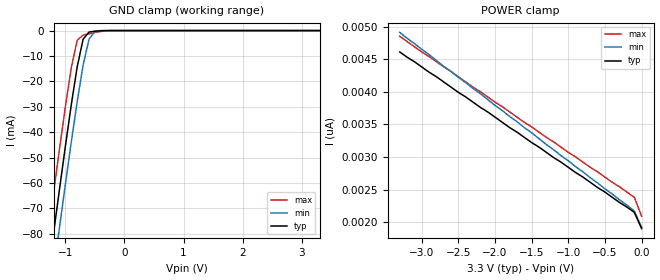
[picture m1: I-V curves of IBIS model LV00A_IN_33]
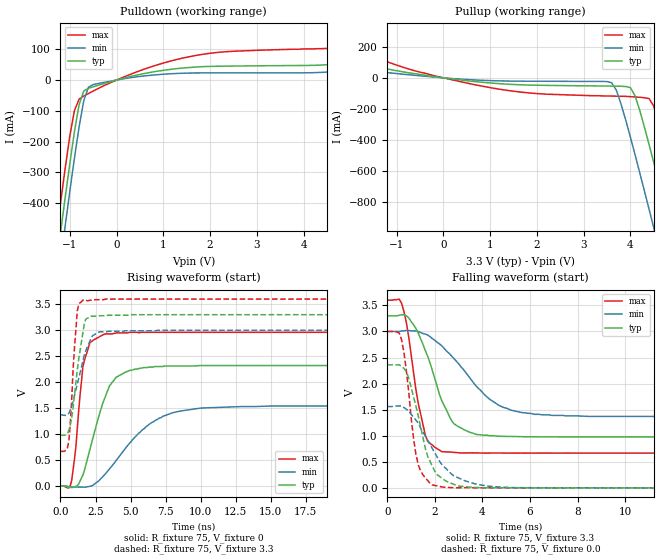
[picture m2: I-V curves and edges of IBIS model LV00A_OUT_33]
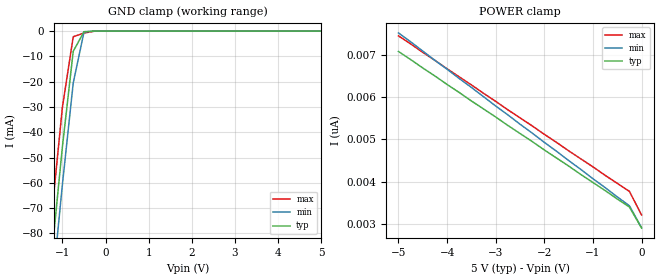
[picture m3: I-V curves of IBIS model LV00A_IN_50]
| TEXAS INSTRUMENTS INCORPORATED
| Standard Linear and Logic Group
| IBIS Model of SN74LV00A
| QUADRUPLE 2-INPUT POSITIVE-NAND GATE
| SOIC 14-pin (D), SOP 14-pin (NS), SSOP 14-pin (DB), TSSOP 14-pin (PW)
| and TVSOP 14-pin (DGV) Package
[IBIS Ver]   3.2
[Comment Char]  |_char
[File Name]   lv00a.ibs
[File Rev]   2.0 I_die
[Date]   May 26, 2000
[Source]   Data created from HSPICE simulations at TI-SLL.
[Notes]   The following is an IBIS list for the LV00A.
|   Please contact sllibis@ti.com with questions and
|   comments concerning SLL IBIS models.
[Disclaimer] Property of Texas Instruments Incorporated.  Unauthorized
   reproduction and/or distribution is strictly prohibited.
   This product is protected under copyright law.
   Created 2000, (C) Copyright 2000, Texas Instruments Inc.,
   All Rights Reserved.
   UNLESS THERE IS A SIGNED, WRITTEN AGREEMENT TO THE
   CONTRARY, TEXAS INSTRUMENTS () IS PROVIDING THE IBIS
   MODELS  AND WITHOUT ANY WARRANTY, EXPRESSED OR
   IMPLIED.  TI assumes no liability for:
   1) the accuracy of the IBIS models provided to your
   company;
   2) the proper functioning of these IBIS Models in your
   design or for any resulting applications; or
   3) infringement of patents, copyrights or intellectual
   property rights resulting from your use of these IBIS
   models.
   TI provides IBIS Models as a service to our customers.
   You and your company shall not distribute, sell or give
   these models to anyone else without prior written
   permission from TI.
   TI reserves the right to make changes to our products or
   to discontinue any semiconductor product or service
   without notice, and advises our customers to obtain the
   latest version of relevant information to verify, before
   placing orders, that the information being relied on is
   current.
   Please be aware that your receipt and use of the IBIS
   information provided shall serve as acceptance of these
   terms and conditions.  If you do not accept these terms,
   you should return or destroy the IBIS models and any
   other accompanying information immediately.
|   Component LV00A_D
[Component]   LV00A_D
[Manufacturer]  Texas Instruments, Inc.
[Package]
|   typ   min   max
R_pkg   0.031   0.028   0.034
L_pkg   3.109nH   2.462nH   3.889nH
C_pkg   0.473pF   0.363pF   0.628pF
[Pin]   signal_name   model_name   R_pin   L_pin   C_pin
1   1A   LV00A_IN   0.033   3.854nH   0.622pF
2   1B   LV00A_IN   0.032   3.188nH   0.473pF
3   1Y   LV00A_OUT   0.028   2.462nH   0.377pF
4   2A   LV00A_IN   0.031   2.596nH   0.363pF
5   2B   LV00A_IN   0.028   2.521nH   0.372pF
6   2Y   LV00A_OUT   0.034   3.250nH   0.476pF
7   GND   GND   0.034   3.889nH   0.628pF
8   3Y   LV00A_OUT   0.034   3.889nH   0.628pF
9   3A   LV00A_IN   0.034   3.250nH   0.476pF
10   3B   LV00A_IN   0.028   2.521nH   0.372pF
11   4Y   LV00A_OUT   0.031   2.596nH   0.364pF
12   4A   LV00A_IN   0.028   2.462nH   0.377pF
13   4B   LV00A_IN   0.032   3.188nH   0.473pF
14   VCC   POWER   0.033   3.854nH   0.622pF
|   Component LV00A_NS
[Component]   LV00A_NS
[Manufacturer]  Texas Instruments, Inc.
[Package]
|   typ   min   max
R_pkg   0.045   0.039   0.054
L_pkg   3.796nH   2.561nH   4.952nH
C_pkg   0.528pF   0.288pF   0.710pF
[Pin]   signal_name   model_name   R_pin   L_pin   C_pin
1   1A   LV00A_IN   0.047   4.867nH   0.706pF
2   1B   LV00A_IN   0.051   4.083nH   0.592pF
3   1Y   LV00A_OUT   0.041   2.915nH   0.376pF
4   2A   LV00A_IN   0.039   2.561nH   0.288pF
5   2B   LV00A_IN   0.041   3.101nH   0.430pF
6   2Y   LV00A_OUT   0.047   4.047nH   0.589pF
7   GND   GND   0.051   4.909nH   0.700pF
8   3Y   LV00A_OUT   0.045   4.784nH   0.694pF
9   3A   LV00A_IN   0.054   4.176nH   0.597pF
10   3B   LV00A_IN   0.039   3.287nH   0.449pF
11   4Y   LV00A_OUT   0.039   2.586nH   0.294pF
12   4A   LV00A_IN   0.040   2.802nH   0.371pF
13   4B   LV00A_IN   0.049   4.080nH   0.593pF
14   VCC   POWER   0.052   4.952nH   0.710pF
|   Component LV00A_DB
[Component]   LV00A_DB
[Manufacturer]  Texas Instruments, Inc.
[Package]
|   typ   min   max
R_pkg   0.044   0.041   0.046
L_pkg   3.551nH   3.258nH   3.927nH
C_pkg   0.402pF   0.360pF   0.421pF
[Pin]   signal_name   model_name   R_pin   L_pin   C_pin
1   1A   LV00A_IN   0.046   3.927nH   0.408pF
2   1B   LV00A_IN   0.044   3.587nH   0.421pF
3   1Y   LV00A_OUT   0.041   3.289nH   0.398pF
4   2A   LV00A_IN   0.042   3.258nH   0.360pF
5   2B   LV00A_IN   0.041   3.286nH   0.403pF
6   2Y   LV00A_OUT   0.044   3.586nH   0.421pF
7   GND   GND   0.046   3.927nH   0.408pF
8   3Y   LV00A_OUT   0.046   3.927nH   0.408pF
9   3A   LV00A_IN   0.044   3.586nH   0.421pF
10   3B   LV00A_IN   0.041   3.286nH   0.403pF
11   4Y   LV00A_OUT   0.043   3.258nH   0.360pF
12   4A   LV00A_IN   0.041   3.289nH   0.398pF
13   4B   LV00A_IN   0.044   3.587nH   0.421pF
14   VCC   POWER   0.046   3.927nH   0.408pF
|   Component LV00A_PW
[Component]   LV00A_PW
[Manufacturer]  Texas Instruments, Inc.
[Package]
|   typ   min   max
R_pkg   0.032   0.029   0.035
L_pkg   2.378nH   2.170nH   2.680nH
C_pkg   0.314pF   0.270pF   0.335pF
[Pin]   signal_name   model_name   R_pin   L_pin   C_pin
1   1A   LV00A_IN   0.033   2.618nH   0.330pF
2   1B   LV00A_IN   0.031   2.313nH   0.317pF
3   1Y   LV00A_OUT   0.030   2.310nH   0.314pF
4   2A   LV00A_IN   0.031   2.173nH   0.272pF
5   2B   LV00A_IN   0.030   2.204nH   0.309pF
6   2Y   LV00A_OUT   0.032   2.315nH   0.317pF
7   GND   GND   0.035   2.680nH   0.335pF
8   3Y   LV00A_OUT   0.033   2.640nH   0.333pF
9   3A   LV00A_IN   0.034   2.347nH   0.319pF
10   3B   LV00A_IN   0.029   2.277nH   0.313pF
11   4Y   LV00A_OUT   0.031   2.170nH   0.270pF
12   4A   LV00A_IN   0.031   2.244nH   0.311pF
13   4B   LV00A_IN   0.033   2.343nH   0.321pF
14   VCC   POWER   0.035   2.657nH   0.332pF
|   Component LV00A_DGV
[Component]   LV00A_DGV
[Manufacturer]  Texas Instruments, Inc.
[Package]
|   typ   min   max
R_pkg   0.035   0.020   0.045
L_pkg   2.499nH   2.077nH   2.966nH
C_pkg   0.361pF   0.305pF   0.416pF
[Pin]   signal_name   model_name   R_pin   L_pin   C_pin
1   1A   LV00A_IN   0.027   2.717nH   0.373pF
2   1B   LV00A_IN   0.037   2.434nH   0.398pF
3   1Y   LV00A_OUT   0.034   2.200nH   0.316pF
4   2A   LV00A_IN   0.020   2.077nH   0.309pF
5   2B   LV00A_IN   0.030   2.147nH   0.305pF
6   2Y   LV00A_OUT   0.042   2.580nH   0.408pF
7   GND   GND   0.039   2.921nH   0.385pF
8   3Y   LV00A_OUT   0.033   2.841nH   0.380pF
9   3A   LV00A_IN   0.042   2.611nH   0.410pF
10   3B   LV00A_IN   0.038   2.331nH   0.329pF
11   4Y   LV00A_OUT   0.026   2.223nH   0.319pF
12   4A   LV00A_IN   0.034   2.259nH   0.313pF
13   4B   LV00A_IN   0.045   2.681nH   0.416pF
14   VCC   POWER   0.042   2.966nH   0.386pF
[Model Selector]   LV00A_IN
LV00A_IN_33   3.3-V Vcc Input Model
LV00A_IN_50   5.0-V Vcc Input Model
[Model Selector]   LV00A_OUT
LV00A_OUT_33   3.3-V Vcc Output Model
LV00A_OUT_50   5.0-V Vcc Output Model
| Models and submodels in the file (4): LV00A_IN_33 (Input), LV00A_OUT_33 (Output), LV00A_IN_50 (Input), LV00A_OUT_50 (Output)
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|   Model LV00A_IN_33
[Model]   LV00A_IN_33
Model_type  Input
Polarity   Inverting
Vinl = 0.99
Vinh = 2.31
| variable   typ   min   max
C_comp   1.24pf   0.94pf   1.54pf
[Temperature Range]   25   85   -40
[Voltage Range]   3.3   3.0   3.6
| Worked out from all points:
|   GND clamp passes 1 mA (typ) near -0.61 V on its own axis
[GND Clamp]
|   Voltage   I(typ)   I(min)   I(max)
-3.3V     -460mA     -475mA     -445mA
-1.3V     -97.5mA    -113mA     -81.5mA
-1.2V     -79.9mA    -95mA      -63.9mA
-1.1V     -62.6mA    -77.6mA    -46.7mA
-1V       -45.6mA    -60.5mA    -30mA
-900mV    -29.2mA    -43.9mA    -14.6mA
-800mV    -14.3mA    -28mA      -3.81mA
-700mV    -3.42mA    -13.6mA    -1.78mA
-600mV    -581uA     -3.4mA     -1.25mA
-500mV    -233uA     -353uA     -759uA
-400mV    -58.1uA    -21.9uA    -324uA
3.3V      1.9nA      2.34nA     1.69nA
[POWER Clamp]
|   Voltage   I(typ)   I(min)   I(max)
-3.3V     4.61nA     4.91nA     4.85nA
-3V       4.38nA     4.65nA     4.61nA
-100mV    2.15nA     2.17nA     2.38nA
0V        1.9nA      1.92nA     2.09nA
|   Model LV00A_OUT_33
[Model]   LV00A_OUT_33
Model_type  Output
Polarity   Non-Inverting
Vmeas = 1.65v
Cref = 15pf
| variable   typ   min   max
C_comp   4.62pf   3.47pf   5.77pf
[Temperature Range]   25   85   -40
[Voltage Range]   3.3   3.0   3.6
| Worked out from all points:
|   slope of the pulldown table from 0 to 0.495 V, typ, clamps not added: 27.3 ohm
|   slope of the pullup table from 0 to 0.495 V, typ, clamps not added: 27.2 ohm
|   rising waveform, R_fixture 75, V_fixture 0: 20-80 % time 1.52ns typ, 3.17ns min, 629ps max; typ from 0 V to 2.32 V
|   falling waveform, R_fixture 75, V_fixture 3.3: 20-80 % time 1.12ns typ, 1.92ns min, 624ps max; typ from 3.3 V to 0.976 V
|   rising waveform, R_fixture 75, V_fixture 3.3: 20-80 % time 664ps typ, 943ps min, 389ps max; typ from 0.976 V to 3.3 V
|   falling waveform, R_fixture 75, V_fixture 0.0: 20-80 % time 811ps typ, 1.31ns min, 468ps max; typ from 2.36 V to 0 V
[Pulldown]
|   Voltage   I(typ)   I(min)   I(max)
-3.3V     -3.04A     -3.13A     -2.95A
-1.3V     -615mA     -707mA     -518mA
-1.2V     -498mA     -591mA     -401mA
-1.1V     -383mA     -475mA     -288mA
-900mV    -167mA     -253mA     -98.6mA
-800mV    -79.1mA    -151mA     -61.7mA
-700mV    -35.5mA    -66.4mA    -51.9mA
-600mV    -26.8mA    -23.2mA    -43.9mA
-500mV    -22mA      -14.7mA    -35.8mA
1.6V      41.2mA     22.8mA     77.1mA
4.7V      52.1mA     27.5mA     106mA
6.6V      86.8mA     47.3mA     166mA
[Pullup]
|   Voltage   I(typ)   I(min)   I(max)
-3.3V     168mA      92.9mA     314mA
600mV     -21.6mA    -12.3mA    -39.7mA
3.6V      -52.9mA    -31.5mA    -117mA
3.8V      -54.2mA    -168mA     -119mA
4V        -62.6mA    -381mA     -121mA
4.1V      -115mA     -494mA     -123mA
4.4V      -429mA     -845mA     -133mA
4.5V      -544mA     -964mA     -182mA
4.8V      -899mA     -1.32A     -505mA
4.9V      -1.02A     -1.44A     -622mA
5.2V      -1.38A     -1.81A     -981mA
6.6V      -3.09A     -3.52A     -2.69A
[Ramp]
| variable   typ   min   max
dV/dt_r   1.39E+00/1.49E-09   9.32E-01/3.20E-09   1.78E+00/6.41E-10
dV/dt_f   1.41E+00/1.08E-09   9.91E-01/1.94E-09   1.77E+00/6.09E-10
R_load = 75
[Rising Waveform]
R_fixture = 75
V_fixture = 0
|   Time   V(typ)   V(min)   V(max)
0s        0V         0V         0V
800ps     -32.3mV    -18.1mV    101mV
1.6ns     209mV      -24.4mV    2.3V
1.7ns     290mV      -25.1mV    2.41V
2.1ns     701mV      -8.51mV    2.76V
3ns       1.58V      173mV      2.91V
3.5ns     1.93V      328mV      2.93V
4.6ns     2.19V      711mV      2.95V
8ns       2.31V      1.41V      2.96V
25ns      2.32V      1.54V      2.96V
[Falling Waveform]
R_fixture = 75
V_fixture = 3.3
V_fixture_min = 3.0
V_fixture_max = 3.6
|   Time   V(typ)   V(min)   V(max)
0s        3.3V       3V         3.6V
600ps     3.32V      3.01V      3.54V
1.1ns     3.13V      3.01V      2.22V
1.6ns     2.63V      2.95V      1.01V
2.3ns     1.66V      2.72V      693mV
2.8ns     1.23V      2.48V      681mV
3.5ns     1.06V      2.09V      672mV
4.7ns     991mV      1.58V      668mV
6.2ns     980mV      1.41V      666mV
25ns      976mV      1.37V      666mV
[Rising Waveform]
R_fixture = 75
V_fixture = 3.3
V_fixture_min = 3.0
V_fixture_max = 3.6
|   Time   V(typ)   V(min)   V(max)
0s        976mV      1.37V      666mV
600ps     1.07V      1.4V       864mV
800ps     1.31V      1.53V      1.64V
900ps     1.5V       1.62V      2.24V
1.2ns     2.23V      1.96V      3.37V
1.6ns     2.95V      2.41V      3.58V
1.8ns     3.21V      2.6V       3.58V
2.3ns     3.27V      2.9V       3.59V
2.8ns     3.28V      2.97V      3.59V
25ns      3.3V       3V         3.6V
[Falling Waveform]
R_fixture = 75
V_fixture = 0.0
|   Time   V(typ)   V(min)   V(max)
0s        2.36V      1.56V      3V
500ps     2.36V      1.57V      2.97V
600ps     2.33V      1.57V      2.84V
800ps     2.23V      1.51V      2.25V
1.2ns     1.57V      1.3V       650mV
1.6ns     752mV      992mV      193mV
1.9ns     410mV      748mV      55.3mV
2.8ns     66.6mV     231mV      2.1mV
4.7ns     2.69mV     16.1mV     545uV
25ns      9.56uV     0V         13.6uV
|   Model LV00A_IN_50
[Model]   LV00A_IN_50
Model_type  Input
Polarity   Inverting
Vinl = 1.5
Vinh = 3.5
| variable   typ   min   max
C_comp   1.24pf   0.94pf   1.54pf
[Temperature Range]   25   85   -40
[Voltage Range]   5.0   4.5   5.5
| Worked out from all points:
|   GND clamp passes 1 mA (typ) near -0.52 V on its own axis
[GND Clamp]
|   Voltage   I(typ)   I(min)   I(max)
-5V       -773mA     -786mA     -758mA
-1.5V     -133mA     -148mA     -117mA
-1.25V    -88.7mA    -104mA     -72.7mA
-1V       -45.6mA    -60.5mA    -30mA
-750mV    -7.99mA    -20.5mA    -2.23mA
-500mV    -233uA     -353uA     -759uA
-250mV    -2.63nA    -182nA     -26.9uA
5V        2.9nA      3.64nA     2.54nA
[POWER Clamp]
|   Voltage   I(typ)   I(min)   I(max)
-5V       7.08nA     7.52nA     7.45nA
-1.5V     4.37nA     4.5nA      4.73nA
-250mV    3.4nA      3.43nA     3.77nA
0V        2.9nA      2.91nA     3.21nA
